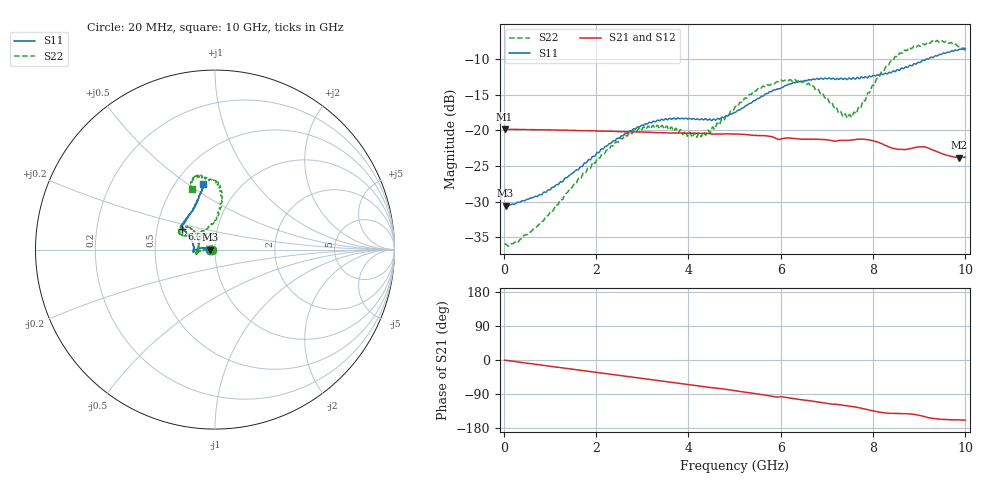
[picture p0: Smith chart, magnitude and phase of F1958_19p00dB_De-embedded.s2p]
! Integrated Device Technology
! Corporate Headquarters
! 6024 Silver Creek Valley Road
! San Jose, CA 95138  USA
! Phone:  1-408-284-8200
! Toll Free:  1-800-223-1366
! Webpage:  http://www.idt.com/
! Timing and RF Division
! 515 Groton Road, Suite 102
! Westford, MA 01886-6024
! Device:  F1958
! Description: 7-bit 0.25 dB Digital Step Attenuator
! Frequency:  0.001 -  6.000 GHz
! Package:  4x4 mm Thin QFN Plastic Package: 24 pin
! Ports:  2 RF, 12 DC
!  Pin  1  = D0
!  Pin  2  = VDD
!  Pin  3  = VMODE
!  Pin  4  = GND
!  Pin  5  = RF1  =  Port 1
!  Pin  6  = GND
!  Pin  7  = GND
!  Pin  8  = GND
!  Pin  9  = GND
!  Pin 10  = GND
!  Pin 11  = GND
!  Pin 12  = GND
!  Pin 13  = GND
!  Pin 14  = RF2  =  Port 2
!  Pin 15  = GND
!  Pin 16  = LE
!  Pin 17  = CLK
!  Pin 18  = DATA
!  Pin 19  = D6
!  Pin 20  = D5
!  Pin 21  = D4
!  Pin 22  = D3
!  Pin 23  = D2
!  Pin 24  = D1
! State:  76
! Atten State:  19.00 dB
! Voltage:  +3.30 Volts
! Current:  0.258 mA
! Data:  The device was measured on a F1958 evaluation board which has
!  individual transmission lines to the RF pins.  Data was collected
!  using a calibrated network analyzer.  The evaluation board was
!  de-embedded using Automatic Fixture Removal (AFR).
!  The reference plane is the edge of the package pin.
! Misc:
!  Action Tracker AT0419
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# GHz S dB R 50
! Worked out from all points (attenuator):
!   500 points, 20 MHz to 10 GHz, reference 50 ohm
!   highest |S21| = -19.85 dB at 20 MHz (marker M1); lowest = -23.8 dB at 9.86 GHz (marker M2)
!   lowest |S11| = -30.6 dB at 40 MHz (marker M3), VSWR 1.06, Z = 47.1 - j0.0405 ohm
!   |S11| at or under -10 dB: start of sweep to 9.207 GHz
!   |S22| runs from -36.2 to -7.4 dB; largest |S21 - S12| = 0.00037
!   S11 on the Smith chart (normalised r, x): 20 MHz: 0.94, -0.00; 6.34 GHz: 0.67, +0.16; 10 GHz: 0.68, +0.58
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0.02  -30.54 -178.9  -19.85 -0.4  -19.85 -0.4  -36.03 -177.1
0.04  -30.57 -179.2  -19.86 -0.8  -19.85 -0.7  -35.94 -175.7
0.32  -30.08 175.1  -19.89 -5.4  -19.89 -5.4  -35.61 -179.7
0.72  -29.28 172.7  -19.92 -11.9  -19.92 -11.9  -33.48 -177.2
1.7  -25.06 171.4  -20.05 -27.7  -20.04 -27.7  -26.31 -178.2
2.6  -20.69 177.5  -20.20 -42.2  -20.18 -42.2  -20.96 -174.5
2.92  -19.53 -178.7  -20.24 -47.4  -20.22 -47.4  -19.74 -171.3
3.36  -18.66 -175.1  -20.34 -54.5  -20.33 -54.6  -19.59 -166.9
4.3  -18.42 -179.1  -20.42 -69.4  -20.43 -69.5  -20.61 164.2
4.64  -18.33 172.3  -20.52 -74.7  -20.54 -74.7  -19.02 151.3
5.02  -17.50 161.2  -20.52 -81.2  -20.52 -81.2  -16.64 139.9
5.56  -15.36 150.7  -20.74 -90.5  -20.76 -90.5  -14.17 140.6
6.34  -13.25 147.9  -21.18 -103.2  -21.19 -103.1  -13.11 154.4
6.68  -12.87 146.7  -21.26 -108.4  -21.28 -108.3  -13.85 154.9
7.3  -12.70 141.0  -21.41 -118.5  -21.43 -118.4  -17.34 134.6
7.5  -12.73 138.4  -21.39 -121.8  -21.39 -121.7  -17.80 115.8
7.68  -12.69 135.5  -21.25 -125.5  -21.26 -125.4  -16.83 98.0
8.34  -11.90 119.3  -22.32 -140.5  -22.33 -140.6  -10.87 82.2
8.68  -11.26 112.6  -22.70 -141.5  -22.70 -141.5  -8.74 86.9
9.26  -9.77 104.9  -22.70 -153.5  -22.69 -153.5  -7.61 100.0
9.86  -8.69 100.0  -23.82 -158.0  -23.84 -157.9  -8.29 109.4
10  -8.55 100.0  -23.77 -158.7  -23.81 -158.6  -8.81 110.4
